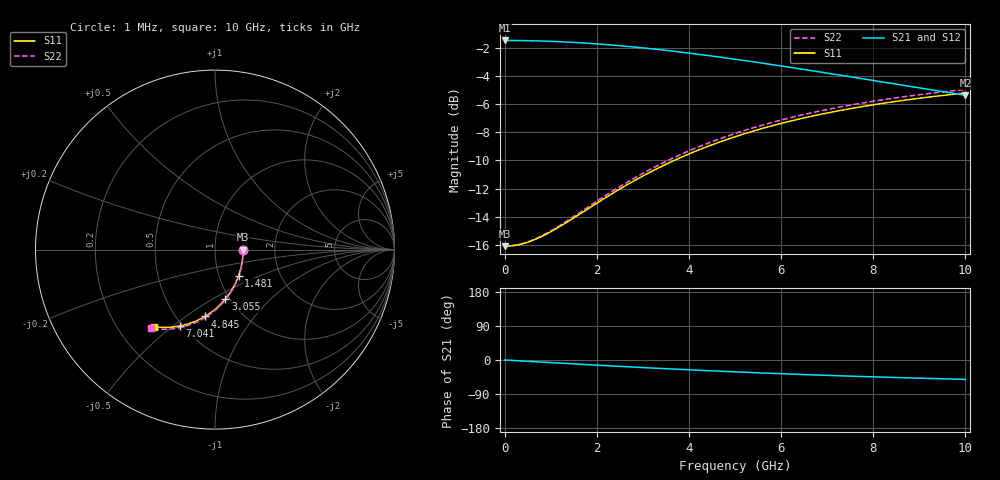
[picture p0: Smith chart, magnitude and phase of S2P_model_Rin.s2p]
! Created Fri Oct 06 13:46:39 2017
# hz S ma R 50
! 2 Port Network Data from SP1.SP block
! freq  magS11  angS11  magS21  angS21  magS12  angS12  magS22  angS22
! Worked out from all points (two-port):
!   10000 points, 1 MHz to 10 GHz, reference 50 ohm
!   highest |S21| = -1.48 dB at 1 MHz (marker M1); lowest = -5.4 dB at 10 GHz (marker M2)
!   |S21| within 3 dB of the highest: start of sweep to 8.308 GHz
!   lowest |S11| = -16.1 dB at 2 MHz (marker M3), VSWR 1.37, Z = 68.6 - j0.0135 ohm
!   |S11| at or under -10 dB: start of sweep to 3.68 GHz
!   |S22| runs from -16.1 to -5.0 dB; largest |S21 - S12| = 0
!   S11 on the Smith chart (normalised r, x): 1 MHz: 1.37, +0.00; 1.481 GHz: 1.24, -0.38; 3.055 GHz: 0.96, -0.57; 4.845 GHz: 0.69, -0.59; 7.041 GHz: 0.49, -0.53; 10 GHz: 0.35, -0.43
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1000000  0.1569 0.0  0.8431 -0.0  0.8431 -0.0  0.1569 0.0
2000000  0.1569 -0.0  0.8431 -0.0  0.8431 -0.0  0.1569 -0.0
1.55e8  0.1574 -5.7  0.8429 -1.1  0.8429 -1.1  0.1575 -5.9
3.08e8  0.1589 -11.3  0.8425 -2.1  0.8425 -2.1  0.159 -11.6
4.67e8  0.1614 -17.1  0.8417 -3.2  0.8417 -3.2  0.1617 -17.5
6.33e8  0.1651 -22.8  0.8407 -4.4  0.8407 -4.4  0.1656 -23.4
9.97e8  0.1764 -34.6  0.8371 -6.9  0.8371 -6.9  0.1776 -35.3
1.481e9  0.1967 -48.1  0.8302 -10.2  0.8302 -10.2  0.1991 -49.0
1.668e9  0.2058 -52.7  0.8268 -11.4  0.8268 -11.4  0.2086 -53.6
2.421e9  0.2459 -68.1  0.8098 -16.3  0.8098 -16.3  0.2507 -68.9
3.055e9  0.2815 -78.2  0.7919 -20.3  0.7919 -20.3  0.2879 -78.9
3.334e9  0.2972 -82.0  0.7831 -22.0  0.7831 -22.0  0.3041 -82.7
4.068e9  0.337 -90.8  0.758 -26.3  0.758 -26.3  0.3456 -91.4
4.845e9  0.3763 -98.4  0.7293 -30.5  0.7293 -30.5  0.3864 -99.0
5.001e9  0.3838 -99.8  0.7233 -31.3  0.7233 -31.3  0.3941 -100.4
5.808e9  0.4199 -106.3  0.692 -35.3  0.692 -35.3  0.4317 -106.8
6.667e9  0.454 -112.2  0.6586 -39.2  0.6586 -39.2  0.467 -112.7
7.041e9  0.4674 -114.5  0.6441 -40.7  0.6441 -40.7  0.4809 -115.0
7.665e9  0.4881 -118.1  0.6205 -43.2  0.6205 -43.2  0.5023 -118.5
8.334e9  0.508 -121.5  0.5959 -45.7  0.5959 -45.7  0.5229 -121.9
9.215e9  0.531 -125.5  0.5649 -48.7  0.5649 -48.7  0.5467 -125.8
1e10  0.5488 -128.6  0.5388 -51.1  0.5388 -51.1  0.5651 -128.9
